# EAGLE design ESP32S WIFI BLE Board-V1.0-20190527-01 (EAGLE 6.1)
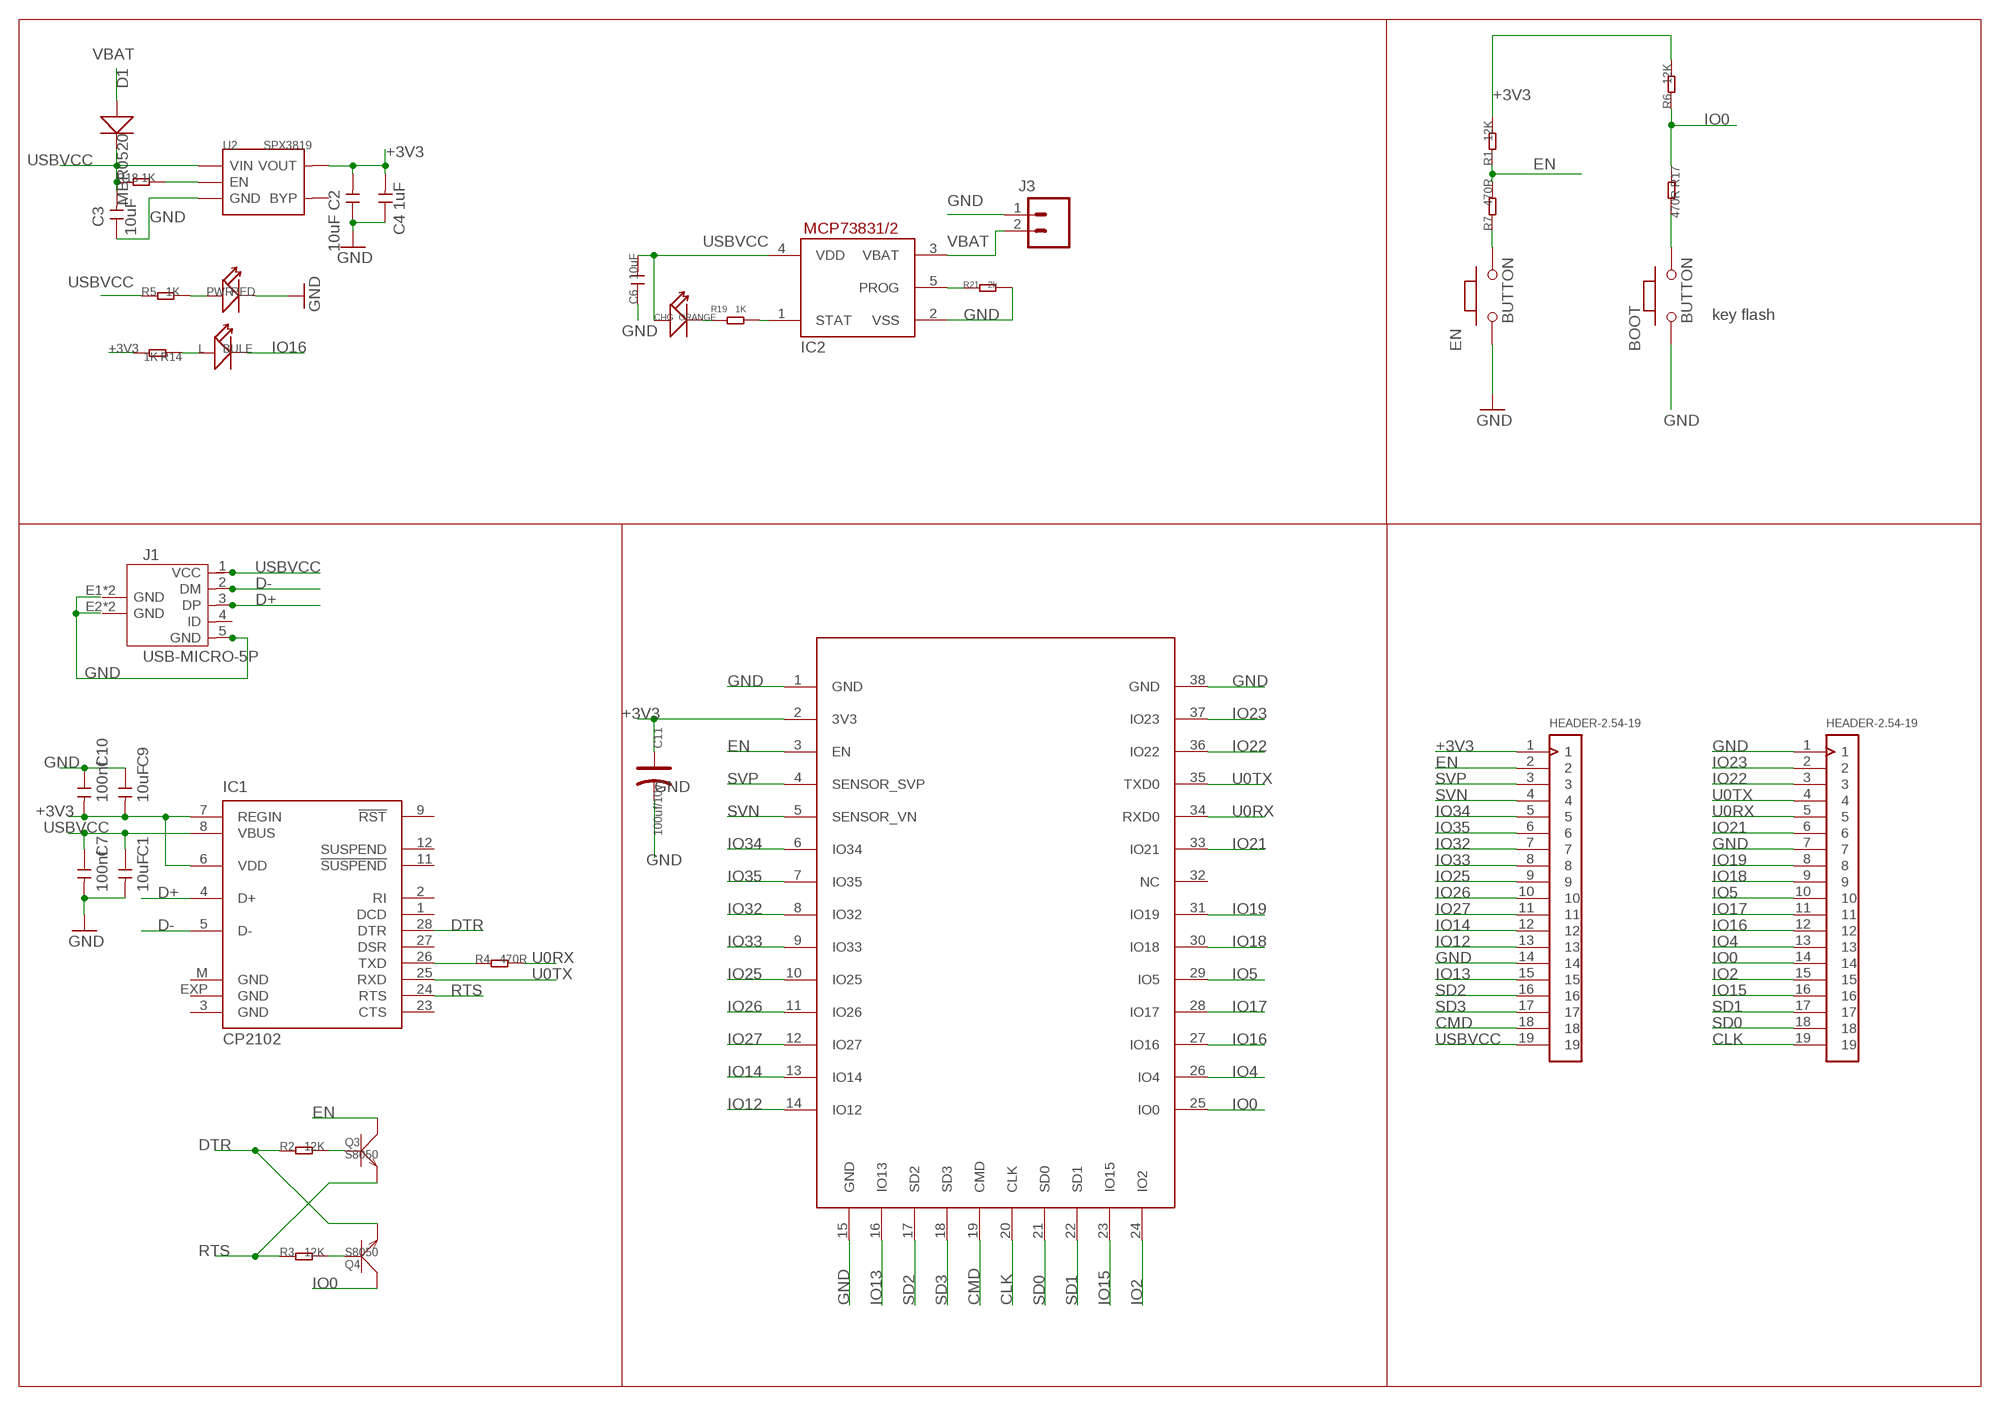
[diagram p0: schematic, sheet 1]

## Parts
BOOT  BUTTON  PB157  [157SW]
C1  10uF  C-0603  [C0603]
C2  10uF  C-0603  [C0603]
C3  10uF  C-0603  [C0603]
C4  1uF  C-0603  [C0603]
C6  10uF  C-0603  [C0603]
C7  100nf  C-0603  [C0603]
C9  10uF  C-0603  [C0603]
C10  100nf  C-0603  [C0603]
C11  100uf/10v  CAP-AVX-B  [AVX-B]
CHG  ORANGE  007-LED0603  [D0603]
D1  MBR0520  D'1206'  [SOD123]
EN  BUTTON  PB157  [157SW]
IC1  CP2102  [MLP28]
IC2  MCP73831/OT  [SOT23-5L]
J1  USB-MICRO-5P  [MICRO-USB-5P]
J3  M02-JST-2MM-SMT  [JST-2-SMD]
L  BULE  LED'0603'  [LED-0603]
PWR  RED  LED'0603'  [LED-0603]
Q3  S8050  TRANSISTOR-NPN-SOT23  [SOT23]
Q4  S8050  TRANSISTOR-NPN-SOT23  [SOT23]
R1  12K  R-0603  [R0603]
R2  12K  R-0603  [R0603]
R3  12K  R-0603  [R0603]
R4  470R  R-0603  [R0603]
R5  1K  R-0603  [R0603]
R6  12K  R-0603  [R0603]
R7  470R  R-0603  [R0603]
R14  1K  R-0603  [R0603]
R17  470R  R-0603  [R0603]
R18  1K  R-0603  [R0603]
R19  1K  R-0603  [R0603]
R21  2k  R-0603  [R0603]
U2  SPX3819  [SOT23-5]
U$1  ESP-32  [ESP-32]
U$3  HEADER-2.54-19  [HEADER-2.54-19]
U$5  HEADER-2.54-19  [HEADER-2.54-19]

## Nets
+3V3: C2.2 C4.2 C9.2 C10.2 C11.+ IC1.6(VDD) IC1.7(REGIN) R1.2 R6.2 R14.2 U2.5(VOUT) U$1.2(3V3) U$3.1
CLK: U$1.20(CLK) U$5.19
CMD: U$1.19(CMD) U$3.18
D+: IC1.4(D+) J1.3(DP)
D-: IC1.5(D-) J1.2(DM)
DTR: IC1.28(DTR) Q4.2(E) R2.1
EN: Q3.3(C) R1.1 R7.2 U$1.3(EN) U$3.2
GND: BOOT.1 C1.2 C2.1 C3.1 C4.1 C6.1 C7.2 C9.1 C10.1 C11.- EN.1 IC2.2(VSS) J1.5(GND) J3.1 PWR.- R21.2 U2.2(GND) U$1.1(GND) U$1.15(GND) U$1.38(GND) U$3.14 U$5.1 U$5.7
IO0: Q4.3(C) R6.1 R17.1 U$1.25(IO0) U$5.14
IO2: U$1.24(IO2) U$5.15
IO4: U$1.26(IO4) U$5.13
IO5: U$1.29(IO5) U$5.10
IO12: U$1.14(IO12) U$3.13
IO13: U$1.16(IO13) U$3.15
IO14: U$1.13(IO14) U$3.12
IO15: U$1.23(IO15) U$5.16
IO16: L.- U$1.27(IO16) U$5.12
IO17: U$1.28(IO17) U$5.11
IO18: U$1.30(IO18) U$5.9
IO19: U$1.31(IO19) U$5.8
IO21: U$1.33(IO21) U$5.6
IO22: U$1.36(IO22) U$5.3
IO23: U$1.37(IO23) U$5.2
IO25: U$1.10(IO25) U$3.9
IO26: U$1.11(IO26) U$3.10
IO27: U$1.12(IO27) U$3.11
IO32: U$1.8(IO32) U$3.7
IO33: U$1.9(IO33) U$3.8
IO34: U$1.6(IO34) U$3.5
IO35: U$1.7(IO35) U$3.6
M8TXD: IC1.26(TXD) R4.1
N$1: CHG.- R19.1
N$2: L.+ R14.1
N$3: PWR.+ R5.2
N$4: EN.2 R7.1
N$5: R18.2 U2.3(EN)
N$8: BOOT.2 R17.2
N$9: Q3.1(B) R2.2
N$10: Q4.1(B) R3.2
N$20: IC2.1(STAT) R19.2
N$31: IC2.5(PROG) R21.1
RTS: IC1.24(RTS) Q3.2(E) R3.1
SD0: U$1.21(SD0) U$5.18
SD1: U$1.22(SD1) U$5.17
SD2: U$1.17(SD2) U$3.16
SD3: U$1.18(SD3) U$3.17
SVN: U$1.5(SENSOR_VN) U$3.4
SVP: U$1.4(SENSOR_SVP) U$3.3
U0RX: R4.2 U$1.34(RXD0) U$5.5
U0TX: IC1.25(RXD) U$1.35(TXD0) U$5.4
USBVCC: C1.1 C3.2 C6.2 C7.1 CHG.+ D1.- IC1.8(VBUS) IC2.4(VDD) J1.1(VCC) R5.1 R18.1 U2.1(VIN) U$3.19
VBAT: D1.+ IC2.3(VBAT) J3.2
Unconnected: IC1.1(DCD) IC1.2(RI) IC1.9(!RST) IC1.11(!SUSPEND) IC1.12(SUSPEND) IC1.23(CTS) IC1.27(DSR) J1.4(ID) J1.E1(GND) J1.E2(GND) J1.P1(GND) J1.P2(GND) U2.4(BYP) U$1.32(NC)

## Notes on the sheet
- 10k=100mA
- 5k=200mA
- 2k=500mA
- 1k=1000mA | key flash

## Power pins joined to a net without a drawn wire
GND: IC1.3(GND) IC1.EXP(GND) IC1.M(GND)

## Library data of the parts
BOOT EN = MySMD:PB157
C1-C4 C6 C7 C9 C10 = Discrete:C*: Ceramic Capacitors
C11 = Discrete:CAP*: Electrolytic Capacitors,Tantalum Capacitors and Super Capacitors
CHG = Discrete:007-LED*
D1 = Discrete:D*
IC1 = silabs:CP210*: Single-Chip USB to UART Bridge Source: www.silabs.com .. CP2101.pdf / cp2102.pdf; MF: FARNELL; MPN: CP2102-GM; OC_FARNELL: 9282130; OC_NEWARK: 30K5635
IC2 = adafruit:MCP73831: MCP73831/2 Miniature Single-Cell, Fully Integrated Li-Ion, Li-Polymer Charge Management Controllers. Nice and small simple lipoly charge controller, with adjustable current and status output (LED) http://www.ladyada.net/library/pcb/eaglelibrary.html
J1 = Connector:USB-MICRO-5P
J3 = SparkFun:M02: Header 2
L PWR = Discrete:LED*
Q3 Q4 = Discrete:TRANSISTOR-NPN*: NPN audion
R1-R7 R14 R17-R19 R21 = Discrete:R*
U2 = IC:SPX3819
U$1 = Discrete:ESP-32
U$3 U$5 = Connector:HEADER-2.54-19

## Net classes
1 power: width 0.61 mm, drill 0.61 mm, clearance 0.254 mm
2 gnd: width 0.305 mm, drill 0.559 mm, clearance 0.254 mm
3 usbvcc: width 0.254 mm, drill 0.61 mm, clearance 0.254 mm
4 aref: width 0.406 mm, drill 0.61 mm, clearance 0.254 mm

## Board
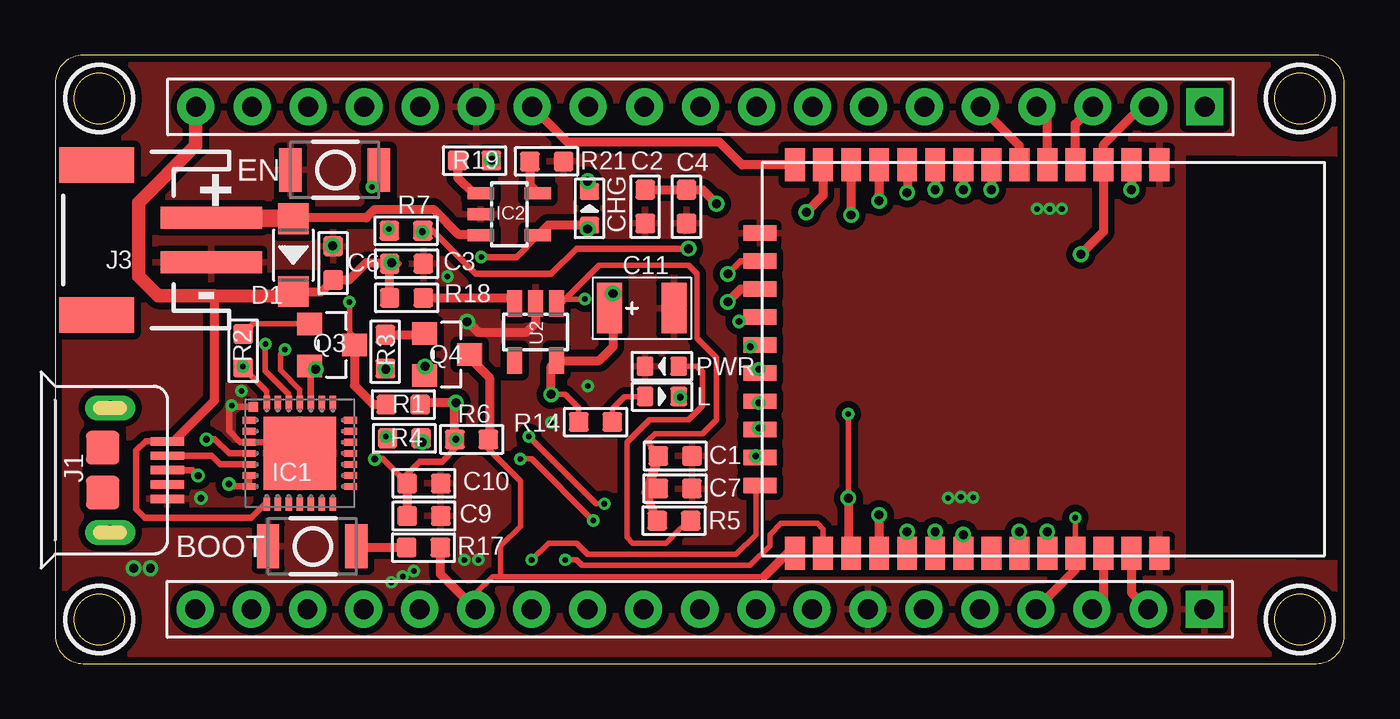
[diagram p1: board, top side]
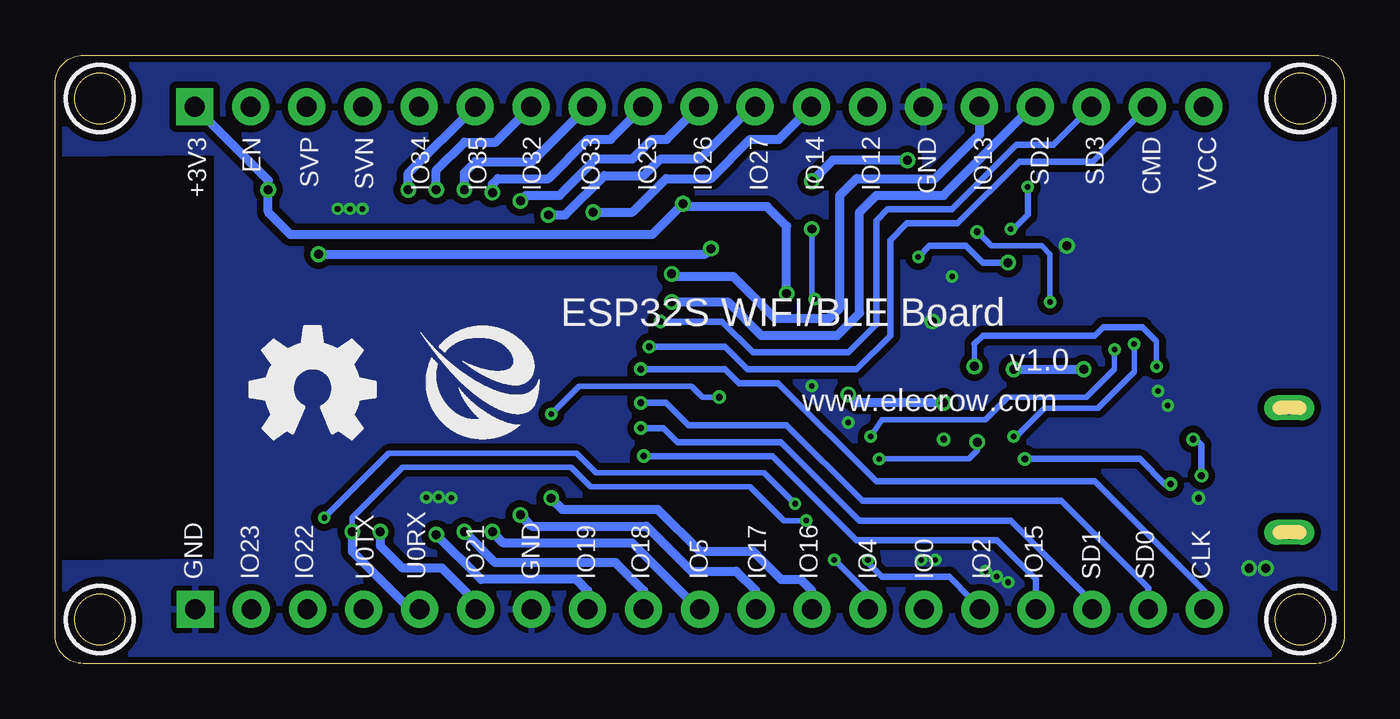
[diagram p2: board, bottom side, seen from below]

Size 58.42 x 27.56 mm. Coordinates in mm from the lower left corner, seen from the top.
Outline: 57.15,27.56 1.27,27.56 arc90 0,26.29 0,1.27 arc90 1.27,0 57.15,0 arc90 58.42,1.27 58.42,26.29 arc90 57.15,27.56
Outline: circle at 56.4,2 radius 1.14
Outline: circle at 56.4,25.6 radius 1.14
Outline: circle at 2,2 radius 1.14
Outline: circle at 2,25.6 radius 1.14
Copper layers (1*16): Top 0.035mm / dielectric 1.5mm / Bottom 0.035mm
Design rules "default": minimum track width 6mil, minimum drill 10mil, track to track 6mil, track to pad 6mil, pad to pad 6mil, via to via 6mil, smd to smd 0mil, copper to edge 10mil, drill to drill 10mil, minimum pad ring 10mil, minimum via ring 6mil, stop-mask expansion 2mil, vias tented up to drill 100mil, thermal gap 10mil
tRestrict: area 54.9,0.5 to 57.9,3.5; area 54.9,24.1 to 57.9,27.1; area 0.5,0.5 to 3.5,3.5; area 0.5,24.1 to 3.5,27.1
bRestrict: area 54.9,0.5 to 57.9,3.5; area 54.9,24.1 to 57.9,27.1; area 0.5,0.5 to 3.5,3.5; area 0.5,24.1 to 3.5,27.1

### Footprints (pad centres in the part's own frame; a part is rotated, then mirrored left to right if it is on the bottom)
157SW = smd 1.016 x 1.981: 1 0,0; 2 4,0
C0603 = smd 0.889 x 0.889: 1 -0.762,0; 2 0.762,0
AVX-B = smd 1.143 x 2.286: + -1.46,0; - 1.46,0
D0603 = smd 0.762 x 0.889: + -0.762,0; - 0.762,0
SOD123 = smd 1.397 x 1.397: + -1.651,0; - 1.651,0
MLP28 = smd 0.6 x 0.3: 1 -2.3,1.5; 2 -2.3,1; 3 -2.3,0.5; 4 -2.3,0; 5 -2.3,-0.5; 6 -2.3,-1; 7 -2.3,-1.5; 15 2.3,-1.5; 16 2.3,-1; 17 2.3,-0.5; 18 2.3,0; 19 2.3,0.5; 20 2.3,1; 21 2.3,1.5 | smd 0.3 x 0.6: 8 -1.5,-2.3; 9 -1,-2.3; 10 -0.5,-2.3; 11 0,-2.3; 12 0.5,-2.3; 13 1,-2.3; 14 1.5,-2.3; 22 1.5,2.3; 23 1,2.3; 24 0.5,2.3; 25 0,2.3; 26 -0.5,2.3; 27 -1,2.3; 28 -1.5,2.3 | smd 3.3 x 3.3: EXP 0,0 | smd 0.435 x 0.435: M -2.103,2.103
SOT23-5L = smd 0.55 x 1.2: 1 -0.95,-1.3; 2 0,-1.3; 3 0.95,-1.3; 4 0.95,1.3; 5 -0.95,1.3
MICRO-USB-5P = smd 0.38 x 1.52: 1 -1.3,0; 2 -0.65,0; 3 0,0; 4 0.65,0; 5 1.3,0 | smd 1.524 x 1.524: E1 -1.016,-2.921; E2 1.016,-2.921 | drill 0.635 pad 1.143 long: P1 -2.819,-2.591; P2 2.819,-2.591
JST-2-SMD = smd 1 x 4.6: 1 -1,-3.7; 2 1,-3.7 | smd 1.6 x 3.4: NC1 -3.4,1.5; NC2 3.4,1.5
LED-0603 = smd 0.762 x 0.889: + -0.762,0; - 0.762,0
SOT23 = smd 1.016 x 1.143: 1 -0.95,-1.016; 2 0.95,-1.016; 3 0,1.016
R0603 = smd 0.889 x 0.889: 1 -0.762,0; 2 0.762,0
SOT23-5 = smd 0.69 x 1.2: 1 -0.95,-1.3; 2 0,-1.3; 3 0.95,-1.3; 4 0.95,1.3; 5 -0.95,1.3
ESP-32 = smd 1.5 x 0.9: 1 -8.8,18.01; 2 -8.8,16.74; 3 -8.8,15.47; 4 -8.8,14.2; 5 -8.8,12.93; 6 -8.8,11.66; 7 -8.8,10.39; 8 -8.8,9.12; 9 -8.8,7.85; 10 -8.8,6.58; 11 -8.8,5.31; 12 -8.8,4.04; 13 -8.8,2.77; 14 -8.8,1.5; 25 8.8,1.5; 26 8.8,2.77; 27 8.8,4.04; 28 8.8,5.31; 29 8.8,6.58; 30 8.8,7.85; 31 8.8,9.12; 32 8.8,10.39; 33 8.8,11.66; 34 8.8,12.93; 35 8.8,14.2; 36 8.8,15.47; 37 8.8,16.74; 38 8.8,18.01 | smd 0.7 x 1.5: 15 -5.71,-0.1; 16 -4.44,-0.1; 17 -3.17,-0.1; 18 -1.9,-0.1; 19 -0.63,-0.1; 20 0.64,-0.1; 21 1.91,-0.1; 22 3.18,-0.1; 23 4.45,-0.1; 24 5.72,-0.1
HEADER-2.54-19 = drill 0.9 pad 1.676 square: 1 0,-25.4 | drill 0.9 pad 1.676: 2 0,-22.86; 3 0,-20.32; 4 0,-17.78; 5 0,-15.24; 6 0,-12.7; 7 0,-10.16; 8 0,-7.62; 9 0,-5.08; 10 0,-2.54; 11 0,0; 12 0,2.54; 13 0,5.08; 14 0,7.62; 15 0,10.16; 16 0,12.7; 17 0,15.24; 18 0,17.78; 19 0,20.32

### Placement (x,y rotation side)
BOOT  9.65,5.31 0 top
C1  28.09,9.4 0 top
C2  26.74,20.7 90 top
C3  15.92,18.11 180 top
C4  28.61,20.7 90 top
C6  12.6,18.14 270 top
C7  28.09,7.93 0 top
C9  16.71,6.68 180 top
C10  16.71,8.16 180 top
C11  26.59,16.1 0 top
CHG  24.21,20.62 90 top
D1  10.79,18.5 270 top
EN  10.67,22.36 0 top
IC1  11.09,9.52 0 top
IC2  20.58,20.35 270 top
J1  5.08,8.76 270 top
J3  3.37,19.19 90 top
L  27.5,12.1 0 top
PWR  27.49,13.47 180 top
Q3  12.55,14.43 270 top
Q4  17.76,13.99 270 top
R1  15.78,11.73 0 top
R2  8.52,14.17 90 top
R3  14.96,14.13 90 top
R4  15.82,10.2 0 top
R5  28.05,6.47 0 top
R6  18.87,10.15 180 top
R7  15.9,19.6 0 top
R14  24.49,10.94 180 top
R17  16.69,5.25 180 top
R18  15.92,16.57 0 top
R19  19,22.78 180 top
R21  22.27,22.75 0 top
U2  21.77,15.02 180 top
U$1  32.03,13.79 270 top
U$2  [OSHW_FILLX200_NOTEXT]  49.59,10.19 0 bottom
U$3  26.7,25.22 90 top
U$4  [ELECROW-NEW]  41.91,10.16 0 bottom
U$5  26.67,2.46 90 top

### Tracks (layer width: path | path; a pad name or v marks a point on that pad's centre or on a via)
+3V3  (via drill 0.3, 0.41)
  Top 0.254: R14.2 23.73,11.58 23.11,12.19 v22.48,12.19
  Top 0.305: IC1.6 IC1.7 7.98,8.02 v7.87,8.13 | v18.16,10.16 R6.2 18.11,9.73 17.53,9.14 16.51,9.14 15.95,8.58 C10.2 14.84,9.27 v14.48,9.27
  Top 0.406: R1.2 16.62,11.81 v18.16,11.81 18.11,11.76 R6.2 | C10.2 C9.2 | U$1.2 v48.77,21.47 v48.77,21.46 | C2.2 C4.2 29.34,21.46 v29.97,20.83 | 25.15,16.97 C11.+ 25.24,16.73 v25.27,16.76 25.27,14.35 24.64,13.72 U2.5 22.48,13.47 v22.48,12.19
  Bottom 0.305: v7.87,8.13 8.13,8.13 9.27,9.27 v14.48,9.27
  Bottom 0.406: U$3.1 48.77,21.89 v48.77,21.46 48.77,20.45 47.75,19.43 31.37,19.43 v29.97,20.83 29.84,20.7 26.16,20.7 25.27,19.81 v25.27,16.76 | v18.16,11.81 22.1,11.81 v22.48,12.19
CLK  (via drill 0.3)
  Top 0.305: U$1.20 31.93,13.13 v31.88,13.34
  Bottom 0.305: U$5.19 6.35,3.3 11.3,8.26 21.21,8.26 25.65,12.7 27.43,12.7 28.07,13.34 v31.88,13.34
CMD  (via drill 0.3)
  Top 0.305: v31.5,14.35 31.86,14.35 U$1.19
  Bottom 0.305: U$3.18 11.4,22.73 14.73,22.73 17.53,19.94 19.81,19.94 20.57,19.18 20.57,14.86 22.1,13.34 27.05,13.34 28.07,14.35 v31.5,14.35
D+  (via drill 0.3)
  Top 0.305: J1.3 6.22,8.76 v6.48,8.51 | IC1.4 7.88,9.52 7.24,10.16 v6.86,10.16
  Bottom 0.305: v6.48,8.51 6.48,9.91 6.73,10.16 v6.86,10.16
D-
  Top 0.305: J1.2 7.1,9.41 7.49,9.02 IC1.5
DTR  (via drill 0.25, 0.41)
  Top 0.254: IC1.28 9.59,12.34 R2.1 8.51,13.4 | Q4.2 16.74,13.44 v16.76,13.46 | v8.51,13.46 8.51,13.4 | 8.51,13.34 8.51,13.4
  Bottom 0.254: v16.76,13.46 16.76,14.48 | 9.14,15.24 8.51,14.61 v8.51,13.46
  Bottom 0.305: 9.14,15.24 10.92,15.24 11.3,14.86 16.38,14.86 16.76,14.48
EN  (via drill 0.25, 0.3, 0.41)
  Top 0.254: 13.59,14.61 13.59,14.73 13.34,14.99 v13.34,16.38
  Top 0.305: R7.2 17.1,19.6 19.05,17.65 22.48,17.65 23.62,18.8 v28.7,18.8
  Top 0.406: U$3.2 49.22,25.22 47.5,23.5 U$1.3 47.5,19.56 v46.48,18.54 | R1.1 14.43,11.73 13.57,12.59 Q3.3 13.57,14.58 13.59,14.61 | v16.64,19.56 16.62,19.56 R7.2
  Bottom 0.254: v13.34,16.38 13.34,18.54 13.72,18.92 16,18.92 v16.64,19.56
  Bottom 0.406: v46.48,18.54 28.96,18.54 v28.7,18.8
GND  (via drill 0.25, 0.3, 0.41)
  Top 0.305: IC1.M 8.06,11.63 v8,11.68 7.87,11.56 7.87,10.54 8.39,10.02 IC1.3 10.59,10.02 IC1.EXP
  Top 0.406: U2.2 21.77,15.42 21.34,14.99 19.18,14.99 v18.67,15.49
  other vias: 3.56,4.32 4.32,4.32 6.6,7.49 8.43,12.34 19.18,4.7 18.54,4.7 15.24,3.68 15.75,3.94 16.26,4.19 17.78,17.53 12.57,18.92 22.48,10.92 24.13,12.57 45.62,20.6 45.06,20.6 44.5,20.6 41.61,7.52 41.05,7.54 40.46,7.49
  pour Top (isolate 0.305, rank 2): -0.1,1.27 -0.1,26.46 arc-90 1.17,27.73 57.25,27.54 arc-90 58.52,26.27 58.52,23.09 51.08,23.16 51.08,4.62 58.77,4.54 58.77,1.27 arc-90 57.5,0 1.17,0 arc-90
  pour Bottom (isolate 0.305, rank 2): 0,1.27 -0.1,26.45 arc-90 1.18,27.73 57.25,27.54 arc-90 58.52,26.27 58.52,23.09 51.08,23.16 51.08,4.62 58.77,4.54 58.77,1.27 arc-90 57.5,0 1.27,0 arc-90
IO0
  Top 0.254: 19.68,10.15 R6.1 19.63,9.7 21.08,8.26 21.08,6.22 20.19,5.33 20.19,3.94 | 32.13,3.94 20.19,3.94 | 20.19,3.94 19.81,3.94 19.05,3.17 U$5.14
  Top 0.406: Q4.3 18.77,13.86 19.68,12.95 19.68,10.2 R6.1 | U$1.25 33.19,4.99 32.13,3.94 | R17.1 17.45,4.06 U$5.14
IO2  (via drill 0.25)
  Top 0.254: v21.59,4.7 22.35,5.46 23.62,5.46 24.13,4.95 30.86,4.95 31.75,5.84 31.75,7.89
  Top 0.305: 31.75,7.89 U$1.24
  Bottom 0.305: v21.59,4.7 21.59,4.57 20.95,3.94 17.91,3.94 16.89,2.92 16.89,2.84 U$5.15
IO4  (via drill 0.25)
  Top 0.254: U$1.26 34.8,6.09 34.54,6.35 32.89,6.35 32.38,5.84 32.38,5.33 31.5,4.45 23.88,4.45 23.62,4.7 v23.11,4.7
  Bottom 0.254: U$5.13 21.59,3.17 v23.11,4.7
IO5  (via drill 0.41)
  Top 0.406: v38.61,5.97 U$1.29
  Bottom 0.406: U$5.10 29.26,2.46 32.26,5.46 38.1,5.46 v38.61,5.97
IO12
  Top 0.406: U$1.14 31.13,22.59 30.1,23.62 23.22,23.62 U$3.13
IO13  (via drill 0.41)
  Top 0.305: U$1.16 31.06,18.23 v30.48,17.65
  Bottom 0.406: U$3.15 16.54,23.98 18.54,21.97 22.1,21.97 22.86,21.21 22.86,16.13 23.37,15.62 25.78,15.62 27.69,17.53 30.35,17.53 v30.48,17.65
IO14  (via drill 0.41)
  Top 0.406: U$1.13 34.8,21.21 v34.04,20.45
  Bottom 0.406: v34.04,20.45 32.26,20.45 30.73,21.97 28.7,21.97 26.92,23.75 25.63,23.75 U$3.12
IO15  (via drill 0.3)
  Top 0.305: U$1.23 31.81,9.34 v31.75,9.4
  Bottom 0.305: U$5.16 13.97,3.81 15.75,5.59 22.1,5.59 25.91,9.4 v31.75,9.4
IO16  (via drill 0.25, 0.3, 0.41)
  Top 0.254: v35.94,11.3 v35.94,7.49
  Top 0.305: L.- 28.42,12.1 v28.32,12.06
  Top 0.406: v35.94,7.49 35.94,5.12 U$1.27
  Bottom 0.254: v28.32,12.06 29.08,12.06 29.59,12.57 34.67,12.57 v35.94,11.3
  Bottom 0.406: v35.94,7.49 35.43,6.99 31.11,6.99 29.21,5.08 26.8,5.08 25.53,3.81 24.64,3.81 24.13,3.3 U$5.12
IO17  (via drill 0.41)
  Top 0.406: v37.34,6.73 U$1.28
  Bottom 0.406: v37.34,6.73 36.83,6.22 31.62,6.22 29.59,4.19 27.56,4.19 26.67,3.3 U$5.11
IO18  (via drill 0.41)
  Top 0.406: v39.88,5.97 U$1.30
  Bottom 0.406: U$5.9 31.75,3.3 33.02,4.57 38.48,4.57 v39.88,5.97
IO19  (via drill 0.41)
  Top 0.406: v41.15,5.84 U$1.31
  Bottom 0.406: U$5.8 34.29,3.3 34.8,3.81 39.12,3.81 v41.15,5.84
IO21  (via drill 0.41)
  Top 0.406: v43.69,5.97 U$1.33
  Bottom 0.406: U$5.6 39.37,2.79 40.89,4.32 42.67,4.32 43.69,5.33 v43.69,5.97
IO22
  Top 0.406: U$1.36 47.5,2.97 U$5.3
IO23
  Top 0.406: U$1.37 48.77,3.22 U$5.2
IO25  (via drill 0.41)
  Top 0.406: U$1.10 v38.61,21.34
  Bottom 0.406: v38.61,21.34 38.61,21.72 38.35,21.97 36.07,21.97 34.29,23.75 33.25,23.75 U$3.9
IO26  (via drill 0.41)
  Top 0.406: U$1.11 v37.34,20.96 v37.34,20.95
  Bottom 0.406: v37.34,20.95 37.08,21.21 35.56,21.21 33.91,22.86 32.26,22.86 31.37,23.75 30.71,23.75 U$3.10
IO27  (via drill 0.41)
  Top 0.406: U$1.12 v36.07,20.32
  Bottom 0.406: v36.07,20.32 35.31,20.32 33.53,22.1 31.75,22.1 30.99,22.86 29.21,22.86 26.85,25.22 U$3.11
IO32  (via drill 0.41)
  Top 0.406: U$1.8 v41.15,21.47 v41.15,21.46
  Bottom 0.406: v41.15,21.46 41.15,22.35 39.88,23.62 38.46,23.62 U$3.7
IO33  (via drill 0.41)
  Top 0.406: U$1.9 v39.88,21.47 v39.88,21.46
  Bottom 0.406: v39.88,21.46 39.88,22.23 39.37,22.73 36.8,22.73 U$3.8
IO34
  Top 0.406: U$1.6 43.69,23.47 U$3.5
IO35  (via drill 0.41)
  Top 0.406: U$1.7 v42.42,21.47 v42.42,21.46
  Bottom 0.406: v42.42,21.46 42.42,22.2 U$3.6
M8TXD  (via drill 0.25)
  Top 0.254: IC1.26 10.59,12.2 9.53,13.26 v9.53,14.48 | v14.99,10.29 14.98,10.29 R4.1
  Bottom 0.254: v9.53,14.48 9.53,13.21 11.18,11.56 13.59,11.56 14.86,10.29 v14.99,10.29
N$1  (via drill 0.41)
  Top 0.406: R19.1 arc45 v19.8,22.8 | v24.13,21.84 24.13,21.46 CHG.-
  Bottom 0.406: v19.8,22.8 23.17,22.8 v24.13,21.84
N$2
  Top 0.254: R14.1 25.25,11.54 25.81,12.1 L.+
N$3
  Top 0.254: R5.2 28.3,6.07 27.69,5.46 26.16,5.46 25.91,5.71 25.91,10.03 26.92,11.05 28.7,11.05 29.34,11.68 29.34,13.21 29.08,13.47 PWR.+
N$4  (via drill 0.25)
  Top 0.254: R7.1 15.14,19.79 v15.11,19.68
  Top 0.305: v14.35,21.59 14.35,22.04 EN.2
  Bottom 0.305: v15.11,19.68 14.99,19.68 14.35,20.32 v14.35,21.59
N$5
  Top 0.406: R18.2 20.58,16.57 U2.3
N$8
  Top 0.406: R17.2 13.71,5.25 BOOT.2
N$9
  Top 0.254: Q3.1 8.97,15.38 R2.2
N$10
  Top 0.406: R3.2 16.69,14.89 Q4.1
N$20
  Top 0.406: IC2.1 18.96,21.3 18.24,22.02 R19.2
N$31
  Top 0.406: R21.1 21.51,21.67 IC2.5
RTS  (via drill 0.41)
  Top 0.305: IC1.24 11.59,13.43 Q3.2
  Top 0.406: R3.1 14.89,13.37 v14.99,13.34 | v11.81,13.34 11.68,13.34 Q3.2
  Bottom 0.406: v14.99,13.34 v11.81,13.34
SD0  (via drill 0.3)
  Top 0.305: v31.88,11.81 31.88,11.83 U$1.21
  Bottom 0.305: U$5.18 8.89,3.43 12.83,7.37 21.84,7.37 25.27,10.79 29.72,10.79 30.73,11.81 v31.88,11.81
SD1  (via drill 0.3)
  Top 0.305: U$1.22 v31.88,10.67
  Bottom 0.305: U$5.17 11.43,2.79 15.11,6.48 21.97,6.48 25.53,10.03 30.23,10.03 30.86,10.67 v31.88,10.67 31.75,10.79
SD2  (via drill 0.41)
  Top 0.406: U$1.17 31.06,16.96 v30.48,16.38
  Bottom 0.406: U$3.16 14.15,25.22 18.16,21.21 21.21,21.21 21.97,20.45 21.97,15.88 22.99,14.86 26.42,14.86 27.94,16.38 v30.48,16.38
SD3  (via drill 0.3)
  Top 0.305: 31.86,15.62 31.11,15.62 v30.99,15.49
  Top 0.406: 31.86,15.62 U$1.18
  Bottom 0.305: U$3.17 13.18,23.5 14.86,23.5 17.78,20.57 20.7,20.57 21.21,20.07 21.21,15.37 22.48,14.1 26.8,14.1 28.19,15.49 v30.99,15.49
SVN
  Top 0.406: U$1.5 44.96,24.74 U$3.4
SVP
  Top 0.406: U$1.4 46.23,24.43 U$3.3
U0RX  (via drill 0.25, 0.41)
  Top 0.254: R4.2 16.59,10.09 v16.64,10.03 | v21.08,9.27 21.59,9.27 v24.38,6.48
  Top 0.406: v44.96,5.97 U$1.34
  Bottom 0.254: v16.64,10.03 16.64,9.65 17.02,9.27 v21.08,9.27 | v44.96,5.97 44.96,6.6 42.67,8.89 35.05,8.89 34.16,8 26.92,8 25.4,6.48 v24.38,6.48
  Bottom 0.406: U$5.5 42.34,2.46 44.96,5.08 v44.96,5.97
U0TX  (via drill 0.25)
  Top 0.254: IC1.25 11.09,12.41 10.21,13.28 10.21,14.02 v10.41,14.22 | v46.23,6.6 U$1.35 | v24.89,7.24 24.51,7.24 v21.46,10.29
  Top 0.406: U$1.35 46.23,4.24 U$5.4
  Bottom 0.254: v10.41,14.22 10.41,13.34 11.68,12.06 15.24,12.06 16.26,11.05 20.95,11.05 v21.46,10.29 | v46.23,6.6 43.31,9.53 34.8,9.53 33.91,8.64 26.29,8.64 v24.89,7.24
USBVCC  (via drill 0.25, 0.41)
  Top 0.254: 23.18,16.57 24.64,18.03 28.7,18.03 29.08,17.65 29.08,14.73 29.97,13.84 29.97,11.05 29.34,10.41 27.18,10.41 26.82,10.06 C1.1 | 23.18,16.57 22.92,16.32 U2.1 | CHG.+ 24.21,19.77 v24.13,19.68 | v24,16.51 23.24,16.51 23.18,16.57
  Top 0.305: IC1.8 9.59,7.3 8.89,6.6 4.06,6.6 3.68,6.99 3.68,9.65 4.09,10.06 J1.1 | C3.2 15.57,18.11 v15.24,18.16 | v19.3,18.41 20.9,18.41 IC2.4
  Top 0.406: C1.1 26.82,7.8 C7.1 26.77,7.75 R5.1 | J1.1 5.36,10.06 7.21,11.91 7.21,16.66 | D1.- 12.07,16.85 C6.2 13.31,17.38 14.1,18.16 15.11,18.16 C3.2 | C3.2 15.16,17.95 15.11,17.91 | R18.1 C3.2 | CHG.+ 22.34,19.86 IC2.4
  Top 0.61: D1.- 10.58,16.64 7.21,16.66 4.67,16.66 3.79,17.55 3.79,20.88 6.38,23.47 U$3.19
  Bottom 0.254: v24.13,19.68 24.13,16.64 v24,16.51
  Bottom 0.305: v15.24,18.16 16.38,18.16 17.14,18.92 18.8,18.92 v19.3,18.41
VBAT
  Top 0.406: 10.29,20.32 10.45,20.15 D1.+ 10.83,20.19 14.1,20.19 14.48,20.57 17.14,20.57 18.29,19.43 19.18,19.43 19.21,19.4 IC2.3
  Top 0.813: D1.+ 7.08,20.18 J3.2

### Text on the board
tPlace: + | -
bNames: VCC | CMD | SD3 | SD2 | IO13 | GND | IO12 | IO14 | IO27 | IO26 | IO25 | IO33 | IO32 | IO35 | IO34 | SVN | SVP | EN | +3V3 | ESP32S WIFI/BLE Board | v1.0 | www.elecrow.com | CLK | SD0 | SD1 | IO15 | IO2 | IO0 | IO4 | IO16 | IO17 | IO5 | IO18 | IO19 | GND | IO21 | U0RX | U0TX | IO22 | IO23 | GND
214bmp: D:/SmartProjects/Snc/a4_bn_logo2.bmp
